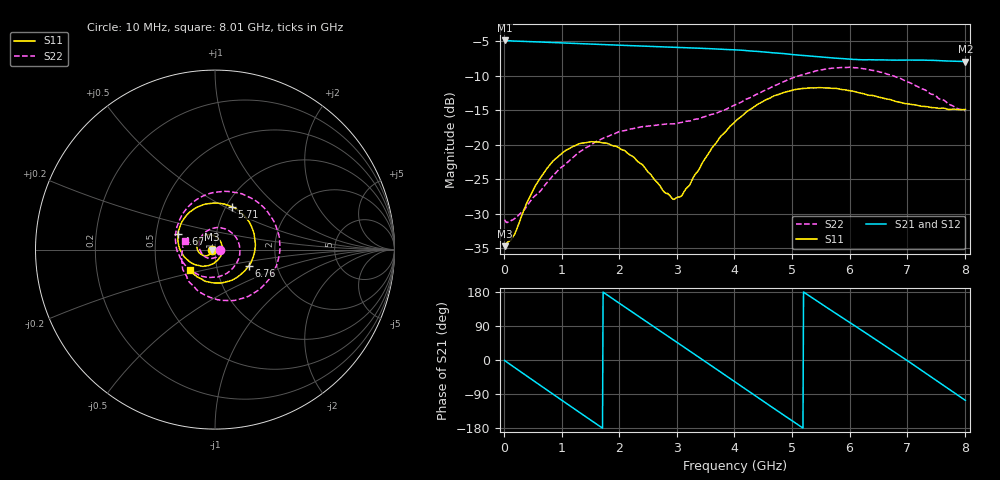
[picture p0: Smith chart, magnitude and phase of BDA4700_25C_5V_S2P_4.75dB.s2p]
!Agilent Technologies,E5071B,MY42404982,A.09.10
!Date: Mon Oct 20 13:28:16 2025
!Data & Calibration Information:
!Freq	S11:SOLT2(ON)	S21:SOLT2(ON)	S12:SOLT2(ON)	S22:SOLT2(ON)
# Hz S RI R 50
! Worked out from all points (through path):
!   801 points, 10 MHz to 8.01 GHz, reference 50 ohm
!   highest |S21| = -4.87 dB at 10 MHz (marker M1); lowest = -7.9 dB at 8.01 GHz (marker M2)
!   group delay of S21, straight-line fit = 286 ps
!   lowest |S11| = -34.7 dB at 10 MHz (marker M3), VSWR 1.04, Z = 48.2 - j0.115 ohm
!   |S11| at or under -10 dB: start of sweep to end of sweep
!   |S22| runs from -31.3 to -8.8 dB; largest |S21 - S12| = 0.0043
!   S11 on the Smith chart (normalised r, x): 10 MHz: 0.96, -0.00; 4.67 GHz: 0.65, +0.12; 5.71 GHz: 1.06, +0.54; 6.76 GHz: 1.44, -0.27; 8.01 GHz: 0.74, -0.17
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1e7  -0.0184 -0.0012  0.5707 -0.0123  0.5707 -0.0129  0.0286 -0.00248
3.3e8  -0.0248 -0.021  0.4585 -0.3253  0.4582 -0.3259  0.0212 -0.0254
7.1e8  -0.0541 -0.0345  0.1399 -0.5367  0.1395 -0.5371  -0.014 -0.0491
1.02e9  -0.0854 -0.0204  -0.1686 -0.5215  -0.1691 -0.5218  -0.0596 -0.0364
1.35e9  -0.1014 0.0168  -0.4287 -0.33  -0.429 -0.3301  -0.0884 0.021
1.93e9  -0.0573 0.0793  -0.4873 0.2043  -0.4872 0.2048  -0.00218 0.1209
2.32e9  -0.00316 0.0756  -0.2357 0.4636  -0.2356 0.4641  0.0999 0.0882
2.68e9  0.0336 0.0397  0.0906 0.5062  0.0907 0.5062  0.1389 -0.0122
2.97e9  0.0403 -0.00567  0.3275 0.3893  0.3276 0.3887  0.1058 -0.0952
3.36e9  0.01 -0.0631  0.4948 0.0844  0.4954 0.0838  0.000435 -0.154
4.01e9  -0.1246 -0.0774  0.2603 -0.4123  0.2607 -0.4123  -0.184 -0.063
4.34e9  -0.1881 -0.0129  -0.0165 -0.4764  -0.0164 -0.4775  -0.2202 0.0549
4.67e9  -0.206 0.0888  -0.2748 -0.3749  -0.2747 -0.3755  -0.1867 0.1885
5.01e9  -0.1556 0.1948  -0.4268 -0.1456  -0.4281 -0.146  -0.0692 0.2974
5.35e9  -0.0462 0.2546  -0.4217 0.1198  -0.4221 0.1191  0.1062 0.3192
5.71e9  0.0921 0.2396  -0.2619 0.3363  -0.2614 0.3364  0.28 0.2258
6.18e9  0.2103 0.1102  0.0643 0.4089  0.0674 0.4095  0.3581 -0.0284
6.68e9  0.2031 -0.0663  0.3533 0.211  0.3542 0.2104  0.2061 -0.2488
6.76e9  0.1893 -0.089  0.379 0.1596  0.38 0.1577  0.1691 -0.2673
7.28e9  0.0507 -0.183  0.354 -0.2084  0.3536 -0.2096  -0.0812 -0.2395
7.65e9  -0.0583 -0.1744  0.1461 -0.3786  0.1448 -0.3797  -0.1807 -0.1046
8.01e9  -0.1401 -0.1137  -0.1147 -0.3848  -0.1145 -0.3853  -0.1696 0.0484
